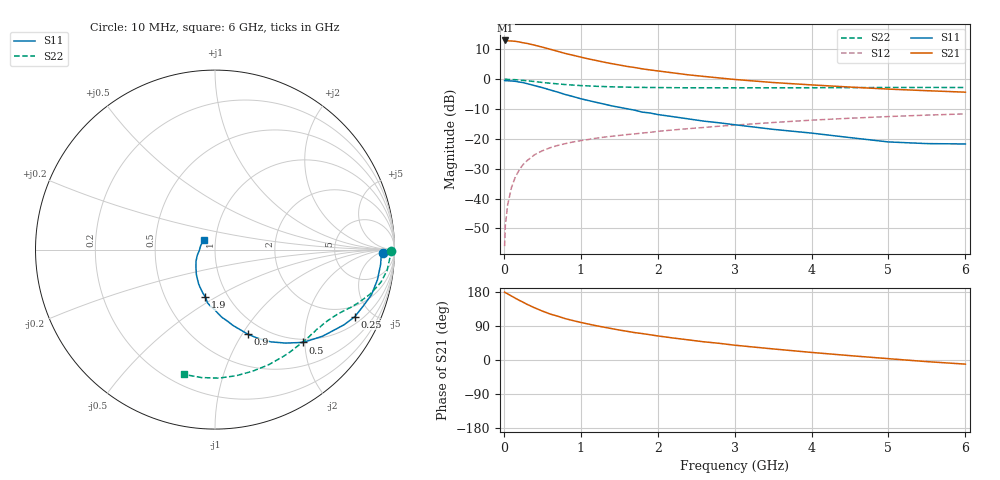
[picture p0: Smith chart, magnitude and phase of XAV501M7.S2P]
! SIEMENS Discrete & RF Semiconductors
! BFY180
! Si NPN RF Bipolar Junction Transistor in MICRO-X
! VCE = 0.5 V  IC = 1.7 mA
! Common Emitter S-Parameters:  May  1997
# GHz  S  MA  R  50
!  f  S11  S21  S12  S22
! GHz  MAG  ANG  MAG  ANG  MAG  ANG  MAG  ANG
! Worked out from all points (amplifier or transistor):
!   36 points, 10 MHz to 6 GHz, reference 50 ohm
!   highest |S21| = 12.8 dB at 20 MHz (marker M1)
!   |S21| within 3 dB of that: start of sweep to 611.4 MHz
!   unconditionally stable (mu >= 1): 1.016 GHz to end of sweep
!   at 250 MHz: K = 0.28, MSG = 20.3 dB, |S12| = -28.6 dB
!   at 1.4 GHz: K = 1.22, MAG = 9.3 dB, |S12| = -19.2 dB
!   at 6 GHz: K = 1.59, MAG = -0.9 dB, |S12| = -11.7 dB
!   S11 on the Smith chart (normalised r, x): 10 MHz: 28, -7; 250 MHz: 1.35, -3.97; 500 MHz: 0.93, -1.96; 900 MHz: 0.84, -1.06; 1.9 GHz: 0.79, -0.45; 6 GHz: 0.88, +0.09
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0.01  0.9351 -1.0  4.298 179.1  0.0016 87.6  0.978 -0.5
0.02  0.9267 -2.1  4.372 177.6  0.0036 87.3  0.9883 -1.0
0.05  0.9264 -5.2  4.311 174.5  0.0079 85.1  0.9768 -2.3
0.1  0.9205 -10.5  4.28 168.8  0.0154 82.5  0.9705 -4.6
0.2  0.8835 -20.9  4.125 157.5  0.03 76.1  0.9533 -9.0
0.25  0.8641 -25.6  3.996 152.5  0.037 72.8  0.9426 -11.0
0.3  0.8315 -30.3  3.908 147.1  0.0427 69.3  0.9277 -12.7
0.4  0.7698 -38.8  3.647 137.7  0.054 64.0  0.8993 -16.0
0.5  0.7129 -46.5  3.384 129.2  0.0627 59.6  0.869 -18.7
0.6  0.653 -52.9  3.124 121.5  0.0705 56.1  0.8447 -21.0
0.7  0.6002 -58.9  2.88 115.6  0.077 52.8  0.8229 -23.0
0.8  0.546 -64.5  2.649 109.1  0.0827 50.8  0.8019 -24.7
0.9  0.5055 -68.8  2.473 104.0  0.0881 48.8  0.7856 -26.3
1.1  0.4332 -76.8  2.151 94.8  0.0969 46.0  0.7604 -29.3
1.5  0.3344 -90.3  1.702 79.1  0.1132 42.0  0.7299 -35.2
1.9  0.2686 -101.6  1.407 66.7  0.1276 39.5  0.7151 -41.0
2.2  0.2329 -109.8  1.257 58.1  0.1398 37.4  0.7107 -45.7
3  0.171 -127.5  0.975 39.1  0.1683 31.9  0.7065 -57.6
3.5  0.1432 -137.9  0.867 29.2  0.1862 28.6  0.7079 -65.2
4.5  0.1042 -161.9  0.728 11.5  0.2195 19.7  0.7125 -80.4
5.5  0.0827 163.7  0.633 -4.3  0.2475 10.6  0.717 -96.1
6  0.0816 141.1  0.598 -10.9  0.2593 5.8  0.7163 -103.9
